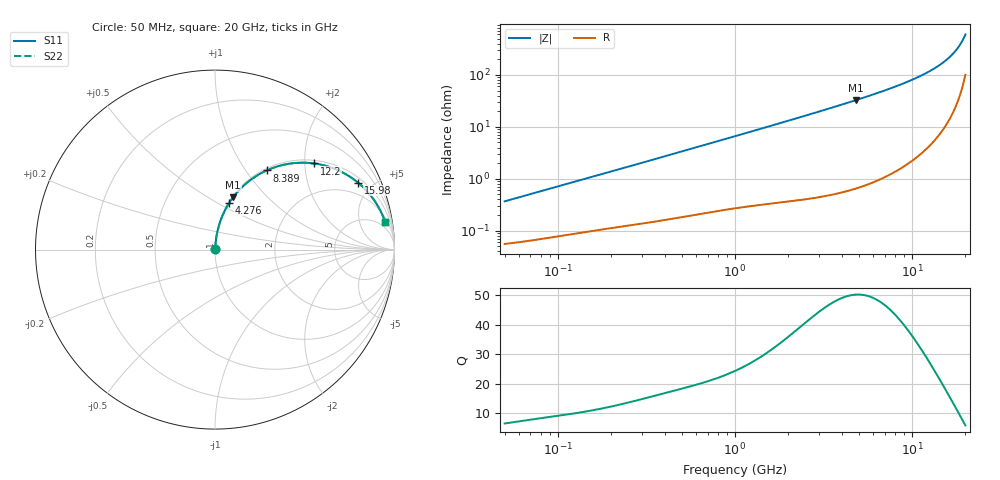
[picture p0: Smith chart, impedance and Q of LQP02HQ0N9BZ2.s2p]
!Murata Part Number: LQP02HQ0N9BZ2
!These Parameters are Measured in Series Mode Connection
!  o--[Z]--o
!Port1  Port2
!  o-------o
!Freq. Start=50[MHz] Stop=20[GHz], 401[Steps]
# Hz S RI R 50
!Freq.(Hz) S11(Real) S11(Imag) S21(Real) S21(Imag) S12(Real) S12(Imag) S22(Real) S22(Imag)
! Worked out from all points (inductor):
!   401 points, 50 MHz to 20 GHz, reference 50 ohm
!   read as one part in series: L = 1.15 nH near 51.52 MHz
!   highest Q = 50.2 at 4.82 GHz (marker M1), where L = 1.08 nH
!   S11 on the Smith chart (normalised r, x): 50 MHz: 1.00, +0.01; 4.276 GHz: 1.01, +0.57; 8.389 GHz: 1.03, +1.26; 12.2 GHz: 1.08, +2.23; 15.98 GHz: 1.25, +4.13; 20 GHz: 3, +12
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5e7  0.000571 0.00363  0.9994 -0.00363  0.9994 -0.00363  0.000571 0.00363
1.364002e8  0.00101 0.00954  0.999 -0.00954  0.999 -0.00954  0.00101 0.00954
3.721004e8  0.00217 0.0251  0.9978 -0.0251  0.9978 -0.0251  0.00217 0.0251
1e9  0.00699 0.0653  0.993 -0.0653  0.993 -0.0653  0.00699 0.0653
1.714689e9  0.0157 0.1102  0.9843 -0.1102  0.9843 -0.1102  0.0157 0.1102
2.728004e9  0.035 0.1724  0.965 -0.1724  0.965 -0.1724  0.035 0.1724
4.275624e9  0.0805 0.2623  0.9195 -0.2623  0.9195 -0.2623  0.0805 0.2623
4.81993e9  0.1011 0.2917  0.8989 -0.2917  0.8989 -0.2917  0.1011 0.2917
6.034176e9  0.1551 0.3519  0.8449 -0.3519  0.8449 -0.3519  0.1551 0.3519
7.442007e9  0.2306 0.4103  0.7694 -0.4103  0.7694 -0.4103  0.2306 0.4103
8.389408e9  0.2882 0.4412  0.7118 -0.4412  0.7118 -0.4412  0.2882 0.4412
9.316812e9  0.3488 0.4639  0.6512 -0.4639  0.6512 -0.4639  0.3488 0.4639
1.034674e10  0.4199 0.4795  0.5801 -0.4795  0.5801 -0.4795  0.4199 0.4795
1.220001e10  0.5521 0.48  0.4479 -0.48  0.4479 -0.48  0.5521 0.48
1.396067e10  0.6741 0.4471  0.3259 -0.4471  0.3259 -0.4471  0.6741 0.4471
1.504638e10  0.7433 0.4116  0.2567 -0.4116  0.2567 -0.4116  0.7433 0.4116
1.597544e10  0.7968 0.3732  0.2032 -0.3732  0.2032 -0.3732  0.7968 0.3732
1.696185e10  0.8467 0.3256  0.1533 -0.3256  0.1533 -0.3256  0.8467 0.3256
1.800918e10  0.8909 0.2691  0.1091 -0.2691  0.1091 -0.2691  0.8909 0.2691
1.855685e10  0.9102 0.2378  0.0898 -0.2378  0.0898 -0.2378  0.9102 0.2378
1.940974e10  0.935 0.1873  0.065 -0.1873  0.065 -0.1873  0.935 0.1873
2e10  0.9484 0.1517  0.0516 -0.1517  0.0516 -0.1517  0.9484 0.1517
